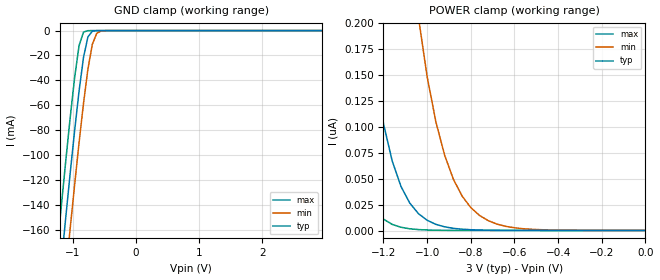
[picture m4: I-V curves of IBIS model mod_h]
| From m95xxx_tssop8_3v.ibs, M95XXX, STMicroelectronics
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|   Model mod_h
[Model]   mod_h
Model_type Input
Vinl   =   0.90V
Vinh   =   2.10V
C_comp   2.120pF   2.024pF   2.323pF
[Temperature Range]  25.0000   85.0000   -40.0000
[Voltage Range]   3.0000V   2.7000V   3.6000V
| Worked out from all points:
|   GND clamp passes 1 mA (typ) near -0.70 V on its own axis
[GND_clamp]
|Voltage   I(typ)   I(min)   I(max)
-3V       -1.187A    -1.23A     -1.145A
-1.25V    -222.4mA   -267.4mA   -176.8mA
-1.18V    -185.7mA   -230.5mA   -140mA
-1.11V    -149.5mA   -194.1mA   -104.1mA
-1.04V    -114.1mA   -158.4mA   -69.45mA
-900mV    -48.41mA   -89.89mA   -11.98mA
-830mV    -21.59mA   -58.45mA   -1.177mA
-760mV    -5.046mA   -30.94mA   -53.02uA
-690mV    -552.5uA   -11.01mA   -2.192uA
-620mV    -47.07uA   -2.191mA   -90.25nA
-550mV    -3.895uA   -303.2uA   -3.716nA
2.95V     6.148pA    45.44pA    6.002pA
[POWER_clamp]
|Voltage   I(typ)   I(min)   I(max)
-3V       4.11uA     3.998uA    5.058uA
-1.44V    753.6nA    1.498uA    266.3nA
-1.4V     579.5nA    1.429uA    172nA
-1.36V    434.3nA    1.333uA    106.3nA
-1.28V    223.8nA    947.4nA    36.16nA
-1.16V    66.83nA    483nA      5.887nA
-1.04V    16.26nA    205.4nA    900.7pA
-920mV    3.548nA    72.52nA    175.6pA
-840mV    1.271nA    33.22nA    89.07pA
-760mV    470.7pA    14.51nA    66.77pA
-560mV    75.45pA    1.728nA    59.57pA
0V        42.97pA    141.4pA    51.35pA
